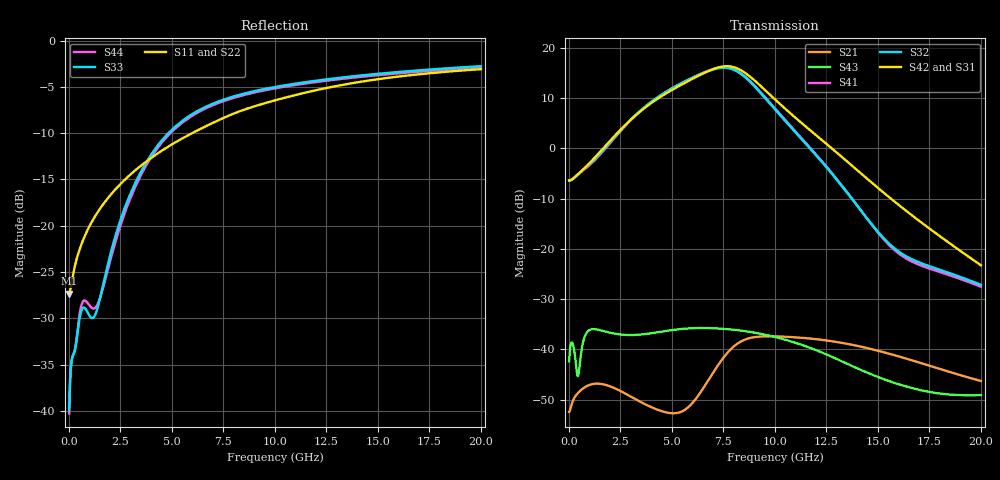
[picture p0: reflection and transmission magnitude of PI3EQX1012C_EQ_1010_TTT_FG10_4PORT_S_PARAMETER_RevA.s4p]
! NPort=4 DATA=2000 NOISE=0 GROUPDELAY=0 COMPLEX_DATAFORMAT=POLAR
! NumOfBlock=1 NumOfParam=0
! .MODEL Smodel S TSTONEFILE=PI3EQX1012C_EQ_1010_TTT_FG10_4PORT_S_PARAMETER_RevA.s4p TYPE=S
!  -- The above .MODEL line can be used for the S element in the netlist.
! The s parameter is extracted from the linear redriver, it is not bi-directional; only s(4,1)s(4,2) and s(3,1)s(3,2)
! should be the insertion loss
!Port definition:
!Port1 = input+
!Port2 = input-
!Port3 = output+
!Port4 = output-
# Hz S MA R  50
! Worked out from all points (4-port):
!   2000 points, 10 MHz to 20 GHz, reference 50 ohm
!   strongest paths, dB at 10 MHz, 5.01 GHz, 10.01 GHz, 15.01 GHz, 20 GHz:
!     S42: -6.4, 11.6, 9.7, -7.9, -23.3
!     S31: -6.4, 11.6, 9.6, -8.1, -23.7
!     S32: -6.4, 11.9, 7.7, -16.7, -27.2
!     S41: -6.4, 11.9, 7.9, -16.8, -27.5
!     S43: -42.4, -36.2, -37.6, -45.5, -49.1
!     S21: -52.4, -52.7, -37.4, -40.3, -46.3
!   lowest |S11| = -27.3 dB at 10 MHz (marker M1), VSWR 1.09, Z = 45.9 - j0.123 ohm
!   |S11| at or under -10 dB: start of sweep to 5.983 GHz
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1e7  0.04301 -178.2  0.002379 1.5  0.0008102 -0.5  0.0008039 -0.5
     0.002388 1.5  0.04109 -178.1  0.000927 -0.5  0.0009197 -0.5
     0.4786 0.1  0.4777 -179.8  0.01016 -4.0  0.007598 -25.7
     0.4772 -179.8  0.4795 0.1  0.007614 -25.8  0.009722 -4.0
4.1e9  0.2368 -124.3  0.002623 1.2  0.0003817 -56.8  0.0003799 -57.2
       0.002605 1.3  0.2405 -123.2  0.0004338 -57.5  0.0004318 -57.8
       2.921 -62.4  3.005 126.8  0.2524 -83.6  0.01361 33.8
       2.992 127.5  2.916 -60.7  0.01455 30.7  0.2446 -83.3
5.79e9  0.3082 -123.7  0.002754 49.9  0.0002762 -58.2  0.000275 -59.2
        0.002651 47.9  0.3132 -123.0  0.0003131 -59.2  0.0003118 -60.2
        4.647 -131.3  4.787 57.5  0.388 -99.8  0.01646 8.8
        4.81 57.7  4.663 -129.4  0.01614 6.2  0.3802 -99.6
7.07e9  0.3629 -124.3  0.006482 65.7  0.0002395 -55.8  0.0002373 -57.1
        0.006158 66.6  0.3683 -123.8  0.0002701 -57.0  0.0002678 -58.4
        6.178 165.3  6.141 -6.7  0.4599 -109.7  0.01673 -11.1
        6.198 -6.8  6.209 167.4  0.01618 -11.9  0.4516 -109.5
8.11e9  0.4079 -125.7  0.01147 44.6  0.0002248 -54.3  0.0002218 -55.8
        0.01113 46.2  0.4138 -125.2  0.000252 -55.6  0.0002487 -57.1
        6.277 101.1  5.901 -71.4  0.5031 -115.9  0.01591 -25.4
        5.975 -71.8  6.311 103.4  0.01558 -25.5  0.4945 -115.8
9.29e9  0.4513 -127.9  0.01361 14.7  0.0002157 -53.8  0.0002118 -55.4
        0.0134 16.2  0.4582 -127.4  0.0002402 -55.0  0.000236 -56.6
        4.176 34.2  3.584 -137.9  0.5414 -121.4  0.01454 -39.6
        3.641 -138.8  4.201 36.8  0.01429 -40.1  0.5327 -121.3
2e10  0.7006 -144.6  0.004898 -74.5  0.0001464 -72.3  0.0001413 -73.8
      0.004848 -73.3  0.7157 -144.4  0.0001623 -72.1  0.0001566 -73.8
      0.06526 102.9  0.0438 29.8  0.7272 -143.5  0.00359 -51.5
      0.04199 28.1  0.0686 107.6  0.003508 -48.8  0.7152 -143.3
